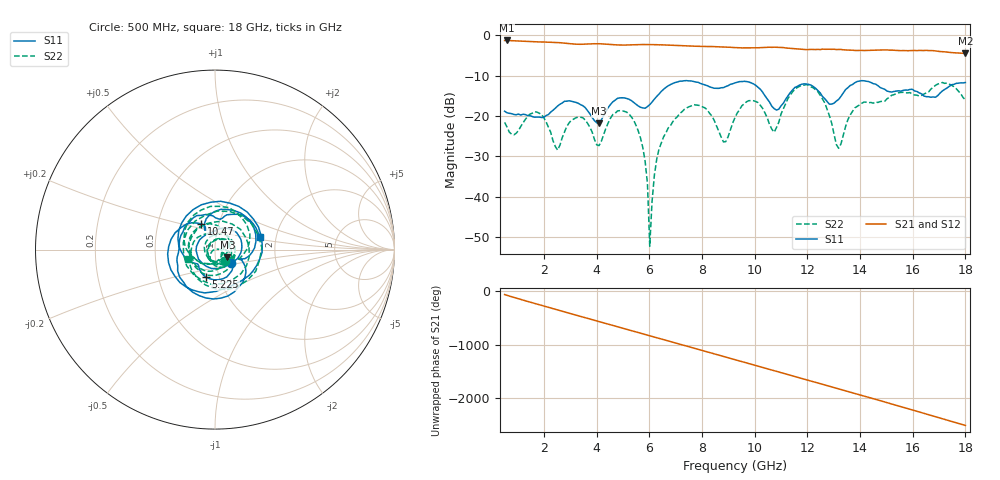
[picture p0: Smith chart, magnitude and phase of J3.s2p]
!Agilent Technologies,N5230A,MY45001360,A.07.50.67
!Agilent N5230A: A.07.50.67
!Date: Tuesday, April 16, 2024 15:51:32
!Correction: S11(Full 2 Port(1,2))
!S21(Full 2 Port(1,2))
!S12(Full 2 Port(1,2))
!S22(Full 2 Port(1,2))
!S2P File: Measurements: S11, S21, S12, S22:
# Hz S  dB  R 50
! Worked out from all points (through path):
!   201 points, 500 MHz to 18 GHz, reference 50 ohm
!   highest |S21| = -1.24 dB at 587.5 MHz (marker M1); lowest = -4.5 dB at 18 GHz (marker M2)
!   group delay of S21, straight-line fit = 388 ps
!   lowest |S11| = -21.7 dB at 4.088 GHz (marker M3), VSWR 1.18, Z = 57.2 - j5.04 ohm
!   |S11| at or under -10 dB: start of sweep to end of sweep
!   |S22| runs from -52.2 to -11.7 dB; largest |S21 - S12| = 0.0077
!   S11 on the Smith chart (normalised r, x): 500 MHz: 1.18, -0.18; 5.225 GHz: 0.87, -0.27; 10.47 GHz: 0.82, +0.24; 18 GHz: 1.65, +0.24
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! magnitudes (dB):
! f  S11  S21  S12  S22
! 500 MHz  -18.8  -1.2  -1.2  -21.5
! 587.5 MHz  -19.1  -1.2  -1.2  -22.6
! 1.812 GHz  -20.2  -1.6  -1.6  -19.3
! 2.513 GHz  -17.5  -1.8  -1.8  -28.4
! 3.475 GHz  -17.4  -2.2  -2.2  -20.4
! 4.088 GHz  -21.7  -2.0  -2.1  -27.3
! 5.225 GHz  -15.8  -2.3  -2.3  -19.5
! 5.838 GHz  -18.0  -2.3  -2.2  -31.2
! 5.925 GHz  -17.6  -2.3  -2.3  -36.7
! 6.013 GHz  -17.1  -2.3  -2.3  -52.2
! 6.188 GHz  -15.8  -2.3  -2.3  -34.7
! 6.362 GHz  -14.5  -2.3  -2.3  -28.2
! 7.675 GHz  -11.4  -2.7  -2.7  -17.1
! 8.812 GHz  -12.9  -2.9  -2.9  -26.4
! 9.25 GHz  -11.8  -3.0  -3.0  -20.3
! 10.47 GHz  -15.7  -2.9  -3.0  -20.4
! 10.74 GHz  -18.1  -2.9  -3.0  -24.0
! 12.22 GHz  -12.7  -3.5  -3.4  -13.0
! 13.19 GHz  -15.8  -3.5  -3.5  -28.0
! 13.8 GHz  -11.7  -3.7  -3.7  -17.9
! 15.11 GHz  -13.9  -3.6  -3.6  -15.3
! 18 GHz  -11.7  -4.5  -4.5  -16.0
